PROGRAM MAIN
VAR
END_VAR


//ACSI Program Code - executes Input Scan, Processing, and Output Scan
 (* ACS_SAMPLE_BACK_AND_FORTH(Axis:=ACS_DRIVES.ACS_DRIVE_1,
	ExtendPosition:=50.0,
	RetractPosition:=5.0,
	ProfileVelocity:=25.0,
	ProfileAccelDecel:=250.0,
	ProfileForce:=100.0); *)
	
(* ACS_SAMPLE_INDEXED_MOVES(Axis := ACS_DRIVES.ACS_DRIVE_1); *)

ACS_SAMPLE_VELOCITY_MOVES(Axis := ACS_DRIVES.ACS_DRIVE_1,
	Speed1 := 20.0,
	Speed2 := 30.0,
	Speed3 := 10.0,
	AccelDecel := 150.0,
	Force := 100.0,
	TimeInSpeedMS := 250);

END_PROGRAM
